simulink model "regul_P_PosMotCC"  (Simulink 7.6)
settings: Solver=ode23t  StartTime=0.0  StopTime=0.6  RelTol=1e-3
InitFcn:
  | close all, clc
  | R1=1e3;
  | R2=0.5e3;
  | C1=1e-3;
  | C2=1e-3;
StopFcn:
  | clc
  | load consigne_position.mat
  | plot(x(1,:),x(2,:),x(1,:),x(3,:))
  | title('Consigne et position de l''arbre moteur')
  | grid
  | %axis([0 1.5e-3 0 2])
  | xlabel('temps')
libraries: fl_lib x18, nesl_utility x5, elec_lib x2

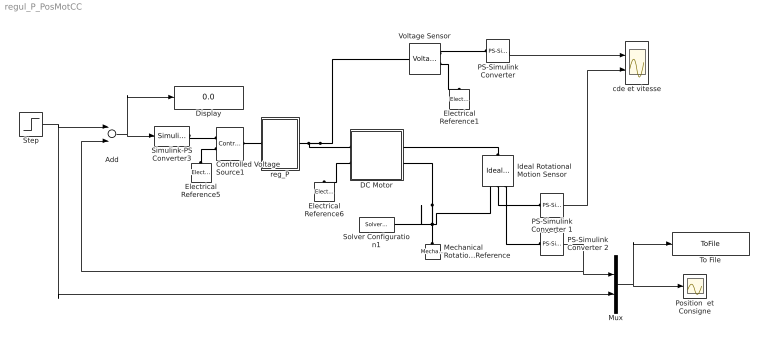
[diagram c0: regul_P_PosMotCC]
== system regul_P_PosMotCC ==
  Add : Sum  Inputs=+-
  Controlled Voltage Source1 : fl_lib/Electrical/Electrical Sources/Controlled Voltage Source  DialogController=NetworkEngine.DynNeDlgSource  SystemSampleTime=-1  i_Log=off  v_Log=off  LocalVarNames=|current|voltage|power  LocalVarDescs=|Current (A)|Voltage (V)|Power (W)  LocalVarLogging=[0 0 0]
  DC Motor : Subsystem
  Display : Display
  Electrical Reference1 : fl_lib/Electrical/Electrical Elements/Electrical Reference  DialogController=NetworkEngine.DynNeDlgSource  SystemSampleTime=-1  i_Log=off  LocalVarNames=|i  LocalVarDescs=|i  LocalVarLogging=[]
  Electrical Reference5 : fl_lib/Electrical/Electrical Elements/Electrical Reference  DialogController=NetworkEngine.DynNeDlgSource  SystemSampleTime=-1  i_Log=off  LocalVarNames=|i  LocalVarDescs=|i  LocalVarLogging=[]
  Electrical Reference6 : fl_lib/Electrical/Electrical Elements/Electrical Reference  DialogController=NetworkEngine.DynNeDlgSource  SystemSampleTime=-1  i_Log=off  LocalVarNames=|i  LocalVarDescs=|i  LocalVarLogging=[]
  Ideal Rotational Motion Sensor : fl_lib/Mechanical/Mechanical Sensors/Ideal Rotational Motion Sensor  DialogController=NetworkEngine.DynNeDlgSource  SystemSampleTime=-1  offset=0 rad  w_Log=off  t_Log=off  phi_Log=off  LocalVarNames=|w|t|phi  LocalVarDescs=|w|t|phi  LocalVarLogging=[]
  Mechanical Rotational Reference : fl_lib/Mechanical/Rotational Elements/Mechanical Rotational Reference  DialogController=NetworkEngine.DynNeDlgSource  SystemSampleTime=-1  t_Log=off  LocalVarNames=|t  LocalVarDescs=|t  LocalVarLogging=[]
  Mux : Mux  Inputs=2
  PS-Simulink Converter : nesl_utility/PS-Simulink Converter  DialogController=NetworkEngine.DynNeUtilDlgSource  SystemSampleTime=-1  PhysicalDomain=network_engine_domain  LeftPortType=input  RightPortType=output  SubClassName=ps_output  Unit=1  AffineConversion=off
  PS-Simulink Converter 1 : nesl_utility/PS-Simulink Converter  DialogController=NetworkEngine.DynNeUtilDlgSource  SystemSampleTime=-1  PhysicalDomain=network_engine_domain  LeftPortType=input  RightPortType=output  SubClassName=ps_output  Unit=1  AffineConversion=off
  PS-Simulink Converter 2 : nesl_utility/PS-Simulink Converter  DialogController=NetworkEngine.DynNeUtilDlgSource  SystemSampleTime=-1  PhysicalDomain=network_engine_domain  LeftPortType=input  RightPortType=output  SubClassName=ps_output  Unit=1  AffineConversion=off
  Position  et Consigne : Scope
  Simulink-PS Converter3 : nesl_utility/Simulink-PS Converter  DialogController=NetworkEngine.DynNeUtilDlgSource  SystemSampleTime=-1  PhysicalDomain=network_engine_domain  LeftPortType=input  RightPortType=output  SubClassName=ps_input  Unit=1  AffineConversion=off  InputFilterTimeConstant=.001  UdotUserProvided=0
  Solver Configuration1 : nesl_utility/Solver Configuration  DialogController=NetworkEngine.DynNeUtilDlgSource  SystemSampleTime=-1  PhysicalDomain=network_engine_domain  LeftPortType=input  RightPortType=generic  SubClassName=solver  Accelerate=off  Profile=off  ResidualTolerance=1e-9  MaxNonlinIter=12  MaxModeIter=2  DoFixedCost=off  UseLocalSampling=off  DoDC=off  LinearAlgebra=Sparse  LocalSolverSampleTime=.001  LocalSolverChoice=NE_BACKWARD_EULER_ADVANCER  UseLocalSolver=off
  Step : Step  Time=0  After=100  SampleTime=0
  To File : ToFile  Filename=consigne_position  MatrixName=x
  Voltage Sensor : fl_lib/Electrical/Electrical Sensors/Voltage Sensor  DialogController=NetworkEngine.DynNeDlgSource  SystemSampleTime=-1  i1_Log=off  v1_Log=off  LocalVarNames=|i1|v1  LocalVarDescs=|i1|v1  LocalVarLogging=[0 0]
  cde et vitesse : Scope  NumInputPorts=2
  reg_P : Subsystem
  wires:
  PS-Simulink Converter 2/1 -> Add/2, Mux/1
  Step/1 -> Add/1, Mux/2
  Mux/1 -> Position  et Consigne/1, To File/1
  PS-Simulink Converter/1 -> cde et vitesse/1
  Add/1 -> Simulink-PS Converter3/1, Display/1
  PS-Simulink Converter 1/1 -> cde et vitesse/2
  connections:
  Electrical Reference5/LConn1 -- Controlled Voltage Source1/RConn2
  Controlled Voltage Source1/LConn1 -- reg_P/LConn1
  DC Motor/LConn2 -- Electrical Reference6/LConn1
  Voltage Sensor/RConn1 -- PS-Simulink Converter/LConn1
  Voltage Sensor/RConn2 -- Electrical Reference1/LConn1
  reg_P/RConn1 -- Voltage Sensor/LConn1 -- DC Motor/LConn1
  Solver Configuration1/RConn1 -- DC Motor/RConn2 -- Mechanical Rotational Reference/LConn1 -- Ideal Rotational Motion Sensor/RConn1
  Simulink-PS Converter3/RConn1 -- Controlled Voltage Source1/RConn1
  Ideal Rotational Motion Sensor/LConn1 -- DC Motor/RConn1
  Ideal Rotational Motion Sensor/RConn3 -- PS-Simulink Converter 2/LConn1
  Ideal Rotational Motion Sensor/RConn2 -- PS-Simulink Converter 1/LConn1

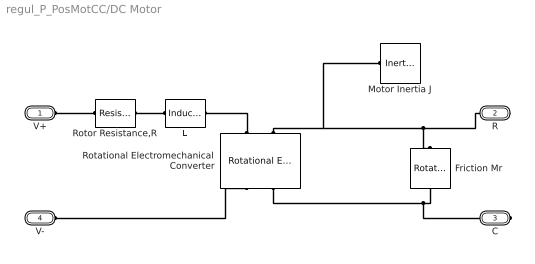
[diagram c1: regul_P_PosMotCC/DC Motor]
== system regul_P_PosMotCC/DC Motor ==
  Friction Mr : fl_lib/Mechanical/Rotational Elements/Rotational Friction  DialogController=NetworkEngine.DynNeDlgSource  SystemSampleTime=-1  brkwy_trq=0.02e-3 N*m  Col_trq=0.02e-3 N*m  visc_coef=0 N*m/(rad/s)  trans_coef=10 s/rad  vel_thr=0.1 rad/s  t_Log=off  w_Log=off  LocalVarNames=|friction_torque|rel_velocity|power  LocalVarDescs=|Friction torque (N*m)|Relative velocity (rad/s)|Power (W)  LocalVarLogging=[0 0 0]
  L : fl_lib/Electrical/Electrical Elements/Inductor  DialogController=NetworkEngine.DynNeDlgSource  SystemSampleTime=-1  l=12e-6 H  i0=0 A  r=0 Ohm  g=1e-09 1/Ohm  i_Log=off  v_Log=off  i_L_Log=off  LocalVarNames=|current|voltage|power  LocalVarDescs=|Inductor current (A) |Voltage across inductor (V)|Power (W)  LocalVarLogging=[0 0 0]
  Motor Inertia J : fl_lib/Mechanical/Rotational Elements/Inertia  DialogController=NetworkEngine.DynNeDlgSource  SystemSampleTime=-1  inertia=0.01 g*cm^2  initial_velocity=0 rad/s  t_Log=off  LocalVarNames=|torque|velocity  LocalVarDescs=|Inertia torque (N*m)|Inertia absolute velocity (rad/s)  LocalVarLogging=[0 0]
  Rotational Electromechanical Converter : fl_lib/Electrical/Electrical Elements/Rotational Electromechanical Converter  DialogController=NetworkEngine.DynNeDlgSource  SystemSampleTime=-1  K=0.072e-3*60/(2*pi) s*V/rad  i_Log=off  v_Log=off  t_Log=off  w_Log=off  LocalVarNames=|current|voltage|power|torque|speed  LocalVarDescs=|Current (A)|Voltage (V)|Power (W)|Torque (Nm)|Angular speed (rad/s)  LocalVarLogging=[0 0 0 0 0]
  Rotor Resistance,R : fl_lib/Electrical/Electrical Elements/Resistor  Tag=Factory Generic  DialogController=NetworkEngine.DynNeDlgSource  SystemSampleTime=-1  R=3.9 Ohm  i_Log=off  v_Log=off  LocalVarNames=|current|voltage|power  LocalVarDescs=|Resistor current (A)|Voltage across resistor (V)|Power (W)  LocalVarLogging=[0 0 0]
  V+ : PMIOPort  Port=1  Side=Left
  R : PMIOPort  Port=2  Side=Right
  C : PMIOPort  Port=3  Side=Right
  V- : PMIOPort  Port=4  Side=Left
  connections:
  Rotational Electromechanical Converter/LConn1 -- L/RConn1
  V-/RConn1 -- Rotational Electromechanical Converter/RConn1
  Rotor Resistance,R/LConn1 -- V+/RConn1
  L/LConn1 -- Rotor Resistance,R/RConn1
  Rotational Electromechanical Converter/LConn2 -- R/RConn1 -- Friction Mr/LConn1 -- Motor Inertia J/LConn1
  Rotational Electromechanical Converter/RConn2 -- C/RConn1 -- Friction Mr/RConn1

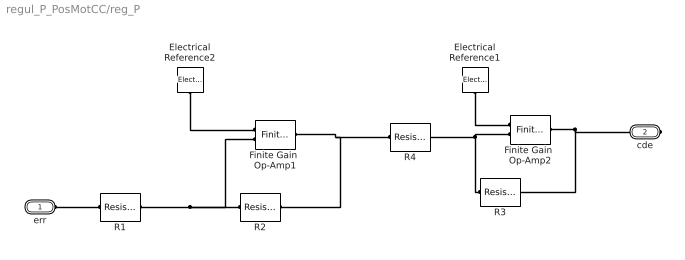
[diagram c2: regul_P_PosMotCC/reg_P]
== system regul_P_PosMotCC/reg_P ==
  Electrical Reference1 : fl_lib/Electrical/Electrical Elements/Electrical Reference  DialogController=NetworkEngine.DynNeDlgSource  SystemSampleTime=-1  i_Log=off  LocalVarNames=|i  LocalVarDescs=|i  LocalVarLogging=[]
  Electrical Reference2 : fl_lib/Electrical/Electrical Elements/Electrical Reference  DialogController=NetworkEngine.DynNeDlgSource  SystemSampleTime=-1  i_Log=off  LocalVarNames=|i  LocalVarDescs=|i  LocalVarLogging=[]
  Finite Gain  Op-Amp1 : elec_lib/Integrated Circuits/Finite Gain Op-Amp  DialogController=NetworkEngine.DynNeDlgSource  SystemSampleTime=-1  A=1000  Rin=1e+6 Ohm  Rout=100 Ohm  Vmin=-15 V  Vmax=15 V  LocalVarLogging=[]
  Finite Gain  Op-Amp2 : elec_lib/Integrated Circuits/Finite Gain Op-Amp  DialogController=NetworkEngine.DynNeDlgSource  SystemSampleTime=-1  A=1000  Rin=1e+6 Ohm  Rout=100 Ohm  Vmin=-15 V  Vmax=15 V  LocalVarLogging=[]
  R1 : fl_lib/Electrical/Electrical Elements/Resistor  DialogController=NetworkEngine.DynNeDlgSource  SystemSampleTime=-1  R=R1 Ohm  i_Log=off  v_Log=off  LocalVarNames=|current|voltage|power  LocalVarDescs=|Resistor current (A)|Voltage across resistor (V)|Power (W)  LocalVarLogging=[0 0 0]
  R2 : fl_lib/Electrical/Electrical Elements/Resistor  DialogController=NetworkEngine.DynNeDlgSource  SystemSampleTime=-1  R=R2 Ohm  i_Log=off  v_Log=off  LocalVarNames=|current|voltage|power  LocalVarDescs=|Resistor current (A)|Voltage across resistor (V)|Power (W)  LocalVarLogging=[0 0 0]
  R3 : fl_lib/Electrical/Electrical Elements/Resistor  DialogController=NetworkEngine.DynNeDlgSource  SystemSampleTime=-1  R=R2 Ohm  i_Log=off  v_Log=off  LocalVarNames=|current|voltage|power  LocalVarDescs=|Resistor current (A)|Voltage across resistor (V)|Power (W)  LocalVarLogging=[0 0 0]
  R4 : fl_lib/Electrical/Electrical Elements/Resistor  DialogController=NetworkEngine.DynNeDlgSource  SystemSampleTime=-1  R=R2 Ohm  i_Log=off  v_Log=off  LocalVarNames=|current|voltage|power  LocalVarDescs=|Resistor current (A)|Voltage across resistor (V)|Power (W)  LocalVarLogging=[0 0 0]
  err : PMIOPort  Port=1  Side=Left
  cde : PMIOPort  Port=2  Side=Right
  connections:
  R3/LConn1 -- Finite Gain  Op-Amp2/LConn2 -- R4/RConn1
  R2/LConn1 -- Finite Gain  Op-Amp1/LConn2 -- R1/RConn1
  R1/LConn1 -- err/RConn1
  Electrical Reference2/LConn1 -- Finite Gain  Op-Amp1/LConn1
  Finite Gain  Op-Amp2/RConn1 -- cde/RConn1 -- R3/RConn1
  R2/RConn1 -- Finite Gain  Op-Amp1/RConn1 -- R4/LConn1
  Electrical Reference1/LConn1 -- Finite Gain  Op-Amp2/LConn1
